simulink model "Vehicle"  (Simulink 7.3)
settings: Solver=ode5  StartTime=0.0  StopTime=200  FixedStep=Ts*2  RelTol=1e-3
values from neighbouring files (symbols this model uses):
  ini = [wbo; atto; Hco]    [start.m]    (also in start1.m; start2.m; start3.m)
  Ixy = 0.476e+7    (= 4760000)    [start.m]
  Ixz = 0.1216e+7    (= 1216000)    [start.m]
  Iyz = 0.30121e+6    (= 301210)    [start.m]
  nt = 12    [start.m]    (also in start1.m; start2.m; start3.m)
  r2d = 180/pi    (= 57.2957795131)    [start.m]    (also in start1.m; start2.m; start3.m)
  wo = 0.0011    [start.m]    (also in start1.m; start2.m; start3.m)
undefined symbols (not defined in the file or in its folder): Av, Bv, CBL, Cv, Dv, Rigbod_Dynam_LVLH

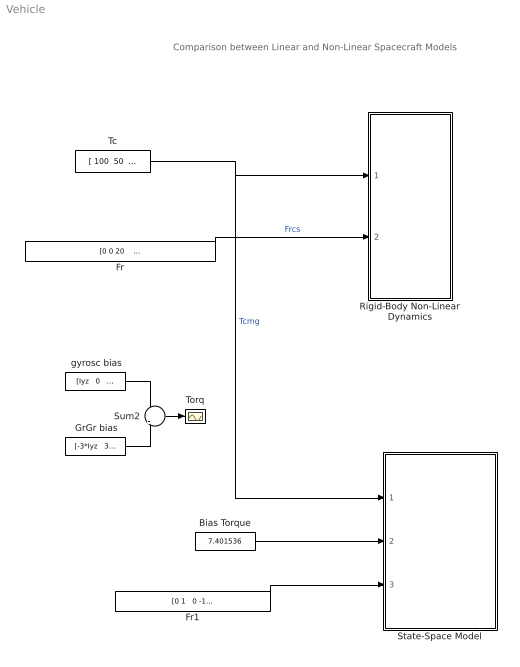
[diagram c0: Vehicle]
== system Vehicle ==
  note: Comparison between Linear and Non-Linear Spacecraft Models
  " GrGr bias" : Constant  Value="[-3*Iyz   3*Ixz    0]' * wo^2"  OutDataType=sfix(16)  OutScaling=2^0
  " gyrosc bias" : Constant  Value="[Iyz   0   -Ixy]' * wo^2"  OutDataType=sfix(16)  OutScaling=2^0
  Bias Torque : Constant  Value=7.401536  OutDataType=sfix(16)  OutScaling=2^0
  Fr : Constant  Value="[0 0 20    0  0 -20    0 0 0    0 0 0]*0"  OutDataType=sfix(16)  OutScaling=2^0
  Fr1 : Constant  Value="[0 1   0 -1   0 0   0 0]*0"  OutDataType=sfix(16)  OutScaling=2^0
  Rigid-Body Non-Linear Dynamics : Subsystem
  State-Space Model : Subsystem
  Sum2 : Sum  Inputs=+|-  OutDataType=sfix(16)  OutScaling=2^0
  Tc : Constant  Value="[ 100  50  10 ]"  OutDataType=sfix(16)  OutScaling=2^0
  Torq : Scope
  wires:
  Tc/1 -> Rigid-Body Non-Linear Dynamics/1(Tc), State-Space Model/1(Tcmg)  "Tcmg"
  Fr1/1 -> State-Space Model/3(Frcs)
  Fr/1 -> Rigid-Body Non-Linear Dynamics/2(f(i))  "Frcs"
  " gyrosc bias"/1 -> Sum2/1
  " GrGr bias"/1 -> Sum2/2
  Sum2/1 -> Torq/1
  Bias Torque/1 -> State-Space Model/2(Tbias)

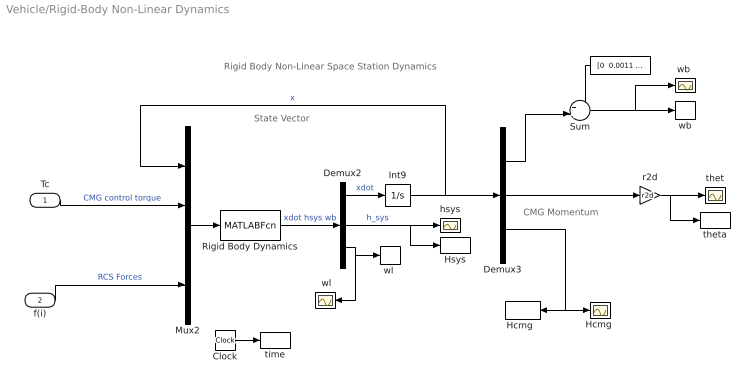
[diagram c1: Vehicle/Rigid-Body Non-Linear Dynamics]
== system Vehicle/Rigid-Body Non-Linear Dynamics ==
  note: Rigid Body Non-Linear Space Station Dynamics
  note: State Vector
  note: CMG Momentum
  Tc : Inport  PortDimensions=3  OutDataType=sfix(16)  OutScaling=2^0
  f(i) : Inport  Port=2  PortDimensions=nt  OutDataType=sfix(16)  OutScaling=2^0
  " " : Constant  Value="[0  0.0011  0]"  OutDataType=sfix(16)  OutScaling=2^0
  " wl" : Scope
  Clock : Clock
  Demux2 : Demux  Outputs=[9,3,3]
  Demux3 : Demux  Outputs=[3,3,3]
  "Hcmg " : Scope
  "Hcmg  " : ToWorkspace  VariableName=Hcmg  SampleTime=-1  SaveFormat=Array
  Hsys : ToWorkspace  VariableName=Hsys  SampleTime=-1  SaveFormat=Array
  Int9 : Integrator  InitialCondition=ini
  Mux2 : Mux  Inputs=[9, 3, 3, nt]
  Rigid Body Dynamics : MATLABFcn  MATLABFcn=Rigbod_Dynam_LVLH( u(1:9), u(10:12), u(13:15), u(16:15+nt) )  OutputDimensions=15
  Sum : Sum  Inputs=++|  OutDataType=sfix(16)  OutScaling=2^0
  hsys : Scope
  r2d : Gain  Gain=r2d  ParameterDataType=sfix(16)  ParameterScaling=2^0  OutDataType=sfix(16)  OutScaling=2^0
  thet : Scope
  theta : ToWorkspace  VariableName=theta  SampleTime=-1  SaveFormat=Array
  time : ToWorkspace  VariableName=time  SampleTime=-1  SaveFormat=Array
  wb : ToWorkspace  VariableName=wb2  SampleTime=-1  SaveFormat=Array
  "wb " : Scope
  "wl " : ToWorkspace  VariableName=wl  SampleTime=-1  SaveFormat=Array
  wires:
  Rigid Body Dynamics/1 -> Demux2/1  "xdot hsys wb"
  Demux2/1 -> Int9/1  "xdot"
  Int9/1 -> Demux3/1, Mux2/1  "x"
  Tc/1 -> Mux2/2  "CMG control torque"
  Demux2/3 -> "wl "/1, " wl"/1
  Demux2/2 -> hsys/1, Hsys/1  "h_sys"
  Demux3/2 -> r2d/1
  Demux3/3 -> "Hcmg  "/1, "Hcmg "/1
  f(i)/1 -> Mux2/4  "RCS Forces"
  r2d/1 -> thet/1, theta/1
  Clock/1 -> time/1
  Mux2/1 -> Rigid Body Dynamics/1
  Sum/1 -> "wb "/1, wb/1
  Demux3/1 -> Sum/2
  " "/1 -> Sum/1

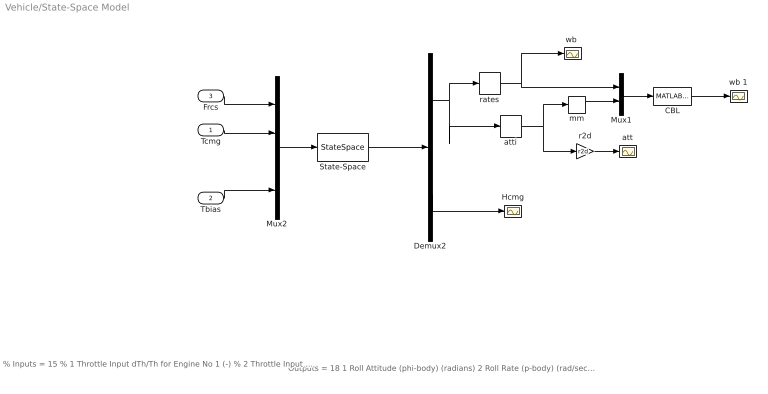
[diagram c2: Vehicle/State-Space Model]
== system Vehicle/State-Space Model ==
  note: Outputs = 18 1 Roll Attitude (phi-body) (radians) 2 Roll Rate (p-body) (rad/sec) 3 Pitch Attitude (thet-bdy) (radians) 4 Pitch Rate (q-body) (rad/sec) 5 Yaw Attitude (psi-body) (radians) 6 Yaw Rate (r-body) (rad/sec) 7 Angle of attack, alfa, (radians) 8 Angle of sideslip, beta, (radian) 9 Change in Altitude, delta-h, (feet) 10 Forward Acceleration (V-dot) (ft/sec) 11 Cross Range Velocity (Vcr) (ft/sec) 12 Accelerom # 1, (along X), (ft/sec^2) Translat. Accelerat. 13 Accelerom # 2, (along Z), (ft/sec^2) Translat. Accelerat. 14 Accelerom # 3, (along X), (ft/sec^2) Translat. Accelerat. 15 Accelerom # 4, (along Z), (ft/sec^2) Translat. Accelerat. 16 Double Gimbal CMG Momentum Change in X-axis (ft-lb-sec) 17 Double Gimbal CMG Momentum Change in Y-axis (ft-lb-sec) 18 Double Gimbal CMG Momentum Change in Z-axis (ft-lb-sec)
  note: % Inputs = 15 % 1 Throttle Input dTh/Th for Engine No 1 (-) % 2 Throttle Input dTh/Th for Engine No 2 (-) % 3 Throttle Input dTh/Th for Engine No 3 (-) % 4 Throttle Input dTh/Th for Engine No 4 (-) % 5 Throttle Input dTh/Th for Engine No 5 (-) % 6 Throttle Input dTh/Th for Engine No 6 (-) % 7 Throttle Input dTh/Th for Engine No 7 (-) % 8 Throttle Input dTh/Th for Engine No 8 (-) % 9 Double Gimbal CMG Torque in the X-axis (ft-lb) % 10 Double Gimbal CMG Torque in the Y-axis (ft-lb) % 11 Double Gimbal CMG Torque in the Z-axis (ft-lb) % 12 Ext Torque Input 1 (ft-lb), dir: 1.00 0.00 0.00 % 13 Ext Torque Input 2 (ft-lb), dir: 0.00 1.00 0.00 % 14 Ext Torque Input 3 (ft-lb), dir: 0.00 0.00 1.00 % 15 Ext Torque Direct.=( 0.1970 -0.5964 -0.7782)
  Tcmg : Inport  PortDimensions=3  OutDataType=sfix(16)  OutScaling=2^0
  Tbias : Inport  Port=2  OutDataType=sfix(16)  OutScaling=2^0
  Frcs : Inport  Port=3  OutDataType=sfix(16)  OutScaling=2^0
  CBL : MATLABFcn  MATLABFcn=CBL( u(1:3), u(4:6) )  OutputDimensions=3
  Demux2 : Demux  Outputs=[11, 4, 3]
  Hcmg : Scope
  Mux1 : Mux  Inputs=[3 , 3]
  Mux2 : Mux  Inputs=[8, 3, 3, 1]
  State-Space : StateSpace  A=Av  B=Bv  C=Cv  D=Dv
  att : Scope
  atti : Selector  InputPortWidth=11  IndexOptions=Index vector (dialog)  Indices=[1 3 5]  OutputSizes=1
  mm : Memory
  r2d : Gain  Gain=r2d  ParameterDataType=sfix(16)  ParameterScaling=2^0  OutDataType=sfix(16)  OutScaling=2^0
  rates : Selector  InputPortWidth=11  IndexOptions=Index vector (dialog)  Indices=[2 4 6]  OutputSizes=1
  "wb " : Scope
  wb 1 : Scope
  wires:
  Mux2/1 -> State-Space/1
  State-Space/1 -> Demux2/1
  Demux2/1 -> rates/1, atti/1
  Frcs/1 -> Mux2/1
  Tcmg/1 -> Mux2/2
  atti/1 -> r2d/1, mm/1
  r2d/1 -> att/1
  rates/1 -> "wb "/1, Mux1/1
  Demux2/3 -> Hcmg/1
  Mux1/1 -> CBL/1
  mm/1 -> Mux1/2
  CBL/1 -> wb 1/1
  Tbias/1 -> Mux2/4
